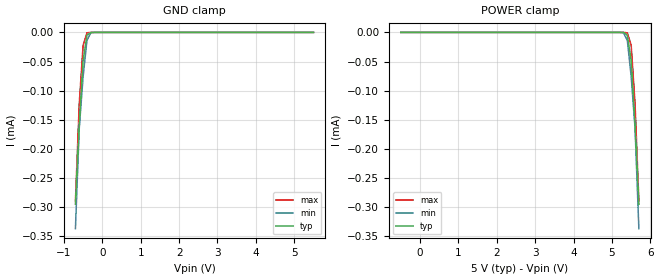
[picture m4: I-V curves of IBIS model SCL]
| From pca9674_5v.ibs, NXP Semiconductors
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[Model]   SCL
Model_type Input
Vinh=3.5
Vinl=1.5
C_comp   5p   4.8p   5.2p
[Model Spec]
Vinh   2.31   1.61   3.85
Vinl   0.99   0.69   1.65
[Temperature Range] 27   85   -40
[Voltage Range]   5   4.5   5.5
[GND Clamp]
-700mV    -295uA     -337uA     -289.5uA
-600mV    -158.8uA   -164.3uA   -122uA
-500mV    -48.62uA   -75.94uA   -22.35uA
-400mV    -4.926uA   -13.83uA   -710.6nA
-300mV    -138.4nA   -722.3nA   -7.551nA
5.5V      13.38pA    37.84pA    11.03pA
[POWER Clamp]
-500mV    13.38pA    37.84pA    11.03pA
5.3V      -138.4nA   -722.3nA   -7.551nA
5.4V      -4.926uA   -13.83uA   -710.6nA
5.5V      -48.62uA   -75.94uA   -22.35uA
5.6V      -158.8uA   -164.3uA   -122uA
5.7V      -295uA     -337uA     -289.5uA
